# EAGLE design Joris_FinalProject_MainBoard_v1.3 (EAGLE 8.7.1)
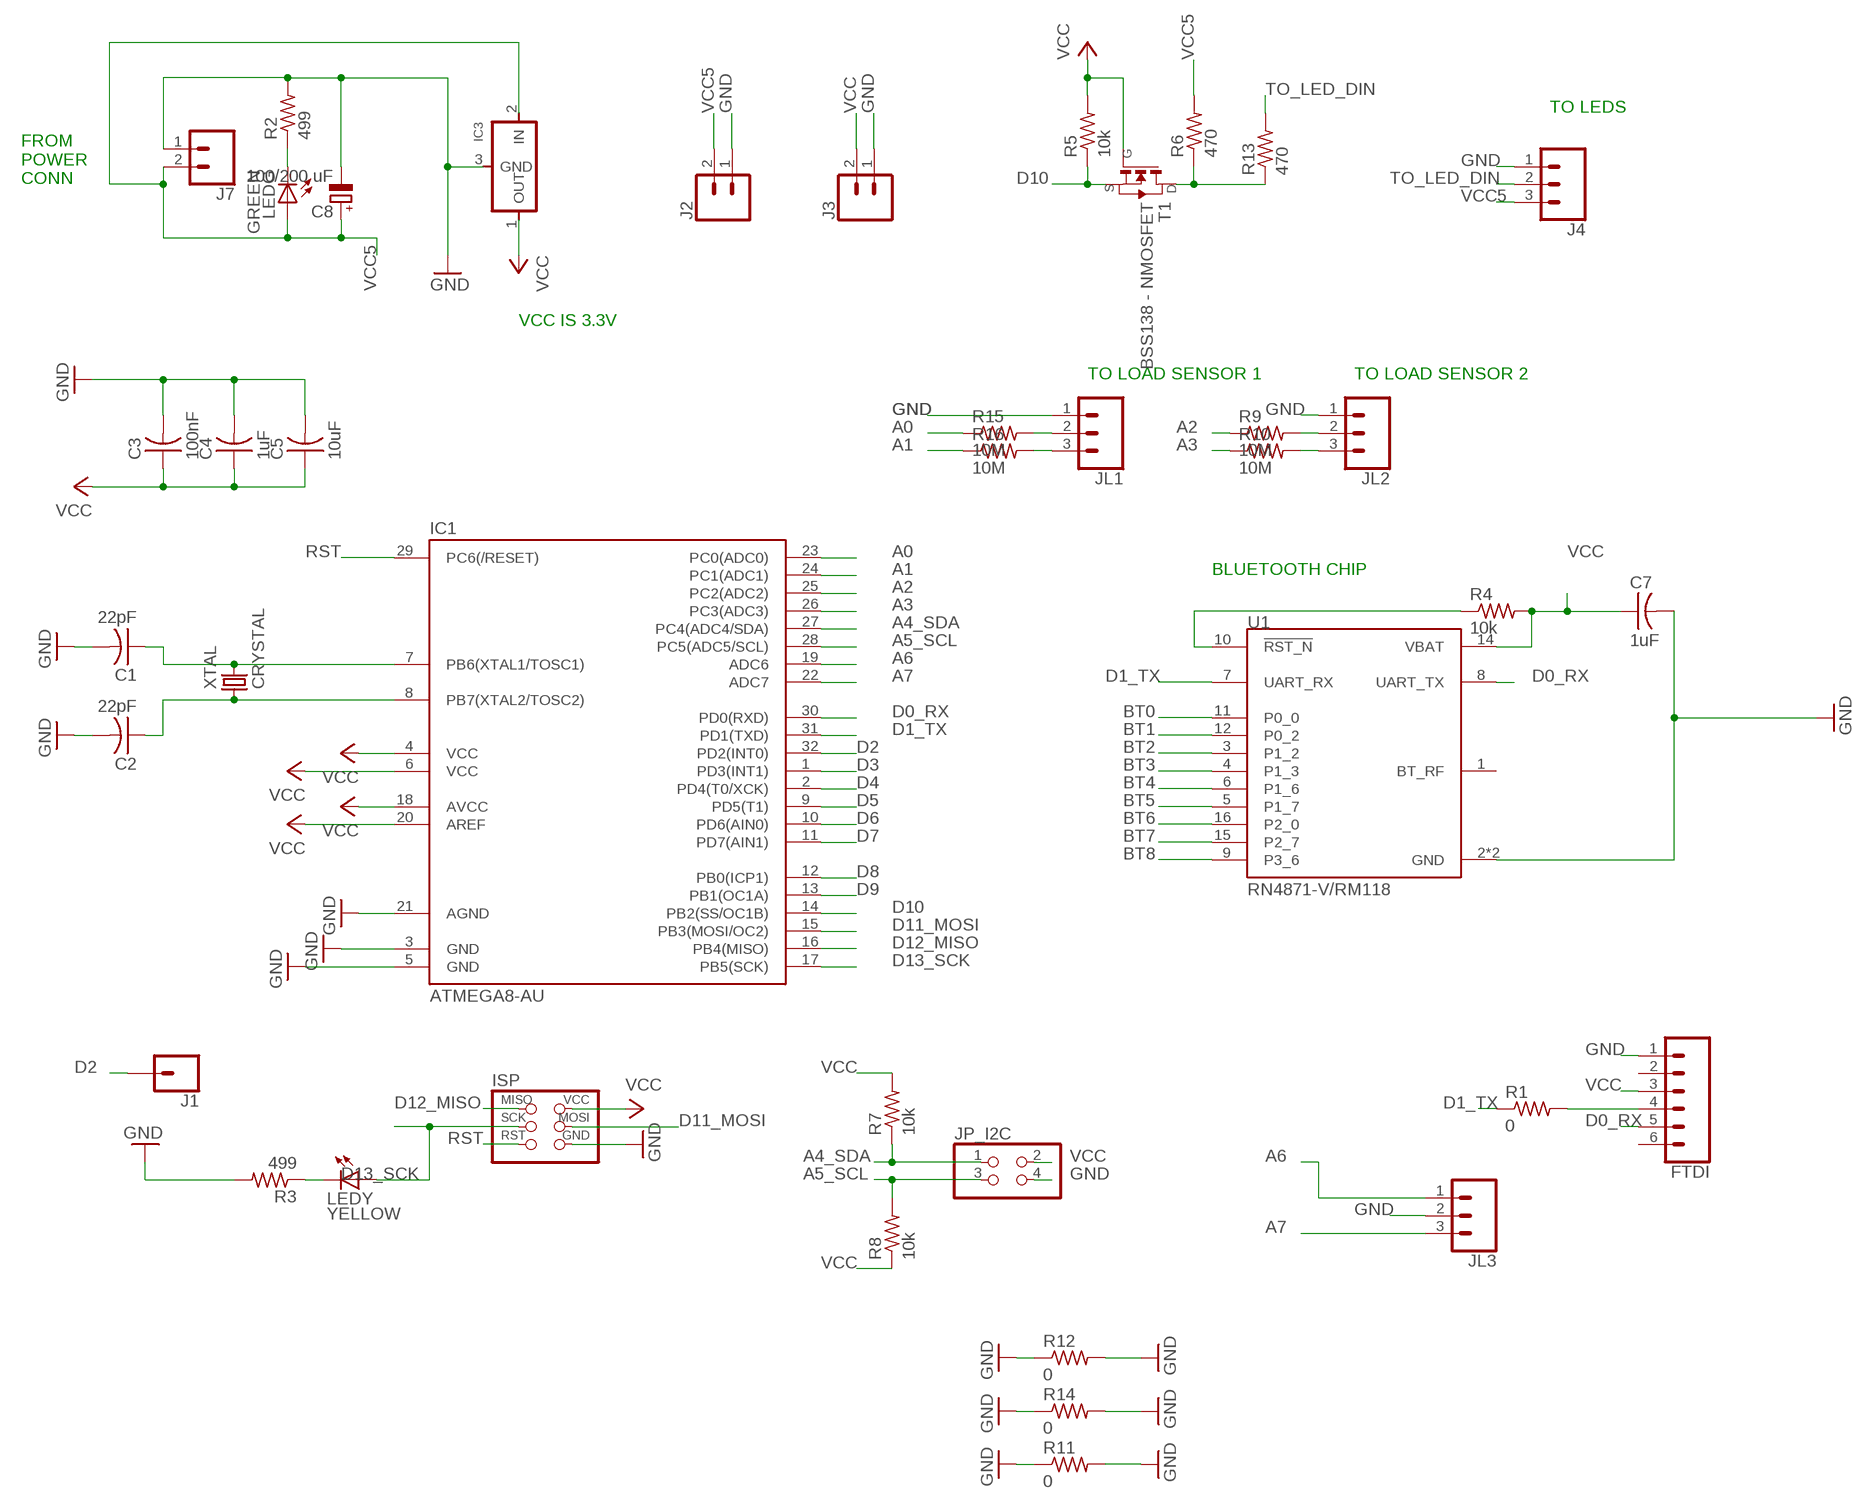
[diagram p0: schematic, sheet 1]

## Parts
C1  22pF  CAP-US1206FAB  [C1206FAB]
C2  22pF  CAP-US1206FAB  [C1206FAB]
C3  100nF  CAP-US1206FAB  [C1206FAB]
C4  1uF  CAP-US1206FAB  [C1206FAB]
C5  10uF  CAP-US1206FAB  [C1206FAB]
C7  1uF  CAP-US1206FAB  [C1206FAB]
C8  100/200 uF  CPOL-EUE3.5-8  [E3,5-8]
FTDI  CONN_06NO_SILK_NO_POP  [1X06_NO_SILK]
IC1  ATMEGA8-AU  [TQFP32-08]
IC3  REGULATORSOT23  [SOT23]
ISP  AVRISPSMD  [2X03SMD]
J1  CONN_01POGOPIN_HOLE_LARGE  [1X01_POGOPIN_HOLE_0.061_DIA]
J2  CONN_02JST-PTH-2  [JST-2-PTH]
J3  CONN_02JST-PTH-2  [JST-2-PTH]
J4  CONN_03JST-PTH-VERT  [JST-3-PTH-VERT]
J7  CONN_02JST-PTH-2  [JST-2-PTH]
JL1  CONN_03JST-PTH-VERT  [JST-3-PTH-VERT]
JL2  CONN_03JST-PTH-VERT  [JST-3-PTH-VERT]
JL3  CONN_03JST-PTH-VERT  [JST-3-PTH-VERT]
JP_I2C  PINHD-2X2-SMD  [2X02SMD]
LEDG  GREEN  LEDFAB1206  [LED1206FAB]
LEDY  YELLOW  LEDFAB1206  [LED1206FAB]
R1  0  RES-US1206FAB  [R1206FAB]
R2  499  RES-US1206FAB  [R1206FAB]
R3  499  RES-US1206FAB  [R1206FAB]
R4  10k  RES-US1206FAB  [R1206FAB]
R5  10k  RES-US1206FAB  [R1206FAB]
R6  470  RES-US1206FAB  [R1206FAB]
R7  10k  RES-US1206FAB  [R1206FAB]
R8  10k  RES-US1206FAB  [R1206FAB]
R9  10M  RES-US1206FAB  [R1206FAB]
R10  10M  RES-US1206FAB  [R1206FAB]
R11  0  RES-US1206FAB  [R1206FAB]
R12  0  RES-US1206FAB  [R1206FAB]
R13  470  RES-US1206FAB  [R1206FAB]
R14  0  RES-US1206FAB  [R1206FAB]
R15  10M  RES-US1206FAB  [R1206FAB]
R16  10M  RES-US1206FAB  [R1206FAB]
T1  BSS138 - NMOSFET  NMOSFETSOT23  [SOT-23]
U1  RN4871-V/RM118  [XCVR_RN4871-V/RM118]
XTAL  CRYSTAL  [2-SMD-5X3MM]

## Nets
A0: IC1.23(PC0(ADC0)) JL1.2 R15.1 R15.2
A1: IC1.24(PC1(ADC1)) JL1.3 R16.1 R16.2
A2: IC1.25(PC2(ADC2)) JL2.2 R9.1 R9.2
A3: IC1.26(PC3(ADC3)) JL2.3 R10.1 R10.2
A4_SDA: IC1.27(PC4(ADC4/SDA)) JP_I2C.1 R7.1
A5_SCL: IC1.28(PC5(ADC5/SCL)) JP_I2C.3 R8.2
A6: IC1.19(ADC6) JL3.1
A7: IC1.22(ADC7) JL3.3
BT0: U1.11(P0_0)
BT1: U1.12(P0_2)
BT2: U1.3(P1_2)
BT3: U1.4(P1_3)
BT4: U1.6(P1_6)
BT5: U1.5(P1_7)
BT6: U1.16(P2_0)
BT7: U1.15(P2_7)
BT8: U1.9(P3_6)
D0_RX: FTDI.5 IC1.30(PD0(RXD)) U1.8(UART_TX)
D1_TX: IC1.31(PD1(TXD)) R1.1 U1.7(UART_RX)
D2: IC1.32(PD2(INT0)) J1.1
D3: IC1.1(PD3(INT1))
D4: IC1.2(PD4(T0/XCK))
D5: IC1.9(PD5(T1))
D6: IC1.10(PD6(AIN0))
D7: IC1.11(PD7(AIN1))
D8: IC1.12(PB0(ICP1))
D9: IC1.13(PB1(OC1A))
D10: IC1.14(PB2(SS/OC1B)) R5.1 T1.2(S)
D11_MOSI: IC1.15(PB3(MOSI/OC2)) ISP.4(MOSI)
D12_MISO: IC1.16(PB4(MISO)) ISP.1(MISO)
D13_SCK: IC1.17(PB5(SCK)) ISP.3(SCK) LEDY.1(A)
GND: C1.2 C2.2 C3.2 C4.2 C5.2 C7.2 C8.- FTDI.1 IC1.3(GND) IC1.5(GND) IC1.21(AGND) IC3.3(GND) ISP.6(GND) J2.1 J3.1 J4.1 J7.1 JL1.1 JL2.1 JL3.2 JP_I2C.4 R2.2 R3.2 R11.1 R11.2 R12.1 R12.2 R14.1 R14.2 U1.2(GND) U1.13(GND)
N$1: LEDY.2(C) R3.1
N$5: LEDG.2(C) R2.1
N$6: C2.1 IC1.8(PB7(XTAL2/TOSC2)) XTAL.P$1
N$7: C1.1 IC1.7(PB6(XTAL1/TOSC1)) XTAL.P$2
N$8: FTDI.4 R1.2
N$12: R4.1 U1.10(!RST_N)
R$4: R6.1 R13.1 T1.1(D)
RST: IC1.29(PC6(/RESET)) ISP.5(RST)
TO_LED_DIN: J4.2 R13.2
VCC: C3.1 C4.1 C5.1 C7.1 FTDI.3 IC1.4(VCC) IC1.6(VCC) IC1.18(AVCC) IC1.20(AREF) IC3.1(OUT) ISP.2(VCC) J3.2 JP_I2C.2 R4.2 R5.2 R7.2 R8.1 T1.3(G) U1.14(VBAT)
VCC5: C8.+ IC3.2(IN) J2.2 J4.3 J7.2 LEDG.1(A) R6.2
Unconnected: FTDI.2 FTDI.6 U1.1(BT_RF)

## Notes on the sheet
- TO LEDS
- FROM
  POWER
  CONN
- VCC IS 3.3V
- TO LOAD SENSOR 1 | TO LOAD SENSOR 2
- BLUETOOTH CHIP

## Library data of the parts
C1-C5 C7 = fab:CAP-US
C8 = rcl:CPOL-EU: POLARIZED CAPACITOR, European symbol; SPICEPREFIX: C
FTDI = SparkFun-Connectors:CONN_06: Multi connection point. Often used as Generic Header-pin footprint for 0.1 inch spaced/style header connections On any of the 0.1 inch spaced packages, you can populate with these: Break Away Headers - Straight (PRT-00116) Break Away Male Headers - Right Angle (PRT-00553) Female Headers (PRT-00115)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
IC1 = atmega8:ATMEGA8
IC3 = fab:REGULATOR
ISP = fab:AVRISP
J1 = SparkFun-Connectors:CONN_01: Single connection point. Often used as Generic Header-pin footprint for 0.1 inch spaced/style header connections
J2 J3 J7 = SparkFun-Connectors_latest:CONN_02: Multi connection point. Often used as Generic Header-pin footprint for 0.1 inch spaced/style header connections; PROD_ID: CONN-09863; SKU: PRT-09914
J4 JL1-JL3 = SparkFun-Connectors_latest:CONN_03: Multi connection point. Often used as Generic Header-pin footprint for 0.1 inch spaced/style header connections On any of the 0.1 inch spaced packages, you can populate with these: Break Away Headers - Straight (PRT-00116) Break Away Male Headers - Right Angle (PRT-00553) Female Headers (PRT-00115)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; PROD_ID: CONN-13230
JP_I2C = fab:PINHD-2X2-SMD
LEDG LEDY = fab:LED: LED
R1-R16 = fab:RES-US: Resistor (US Symbol)
T1 = fab:NMOSFET: MOS FET
U1 = RN4871-V_RM118:RN4871-V/RM118: Bluetooth 4.2 BLE Module Shielded Antenna ASCII Interface 9x11.5mm; AVAILABILITY: Good; DESCRIPTION: Bluetooth 4.2 BLE Module Shielded Antenna ASCII Interface 9x11.5mm; MF: Microchip; MP: RN4871-V/RM118; PACKAGE: SMD-16 Microchip; PRICE: 7.65 USD
XTAL = fab:CRYSTAL

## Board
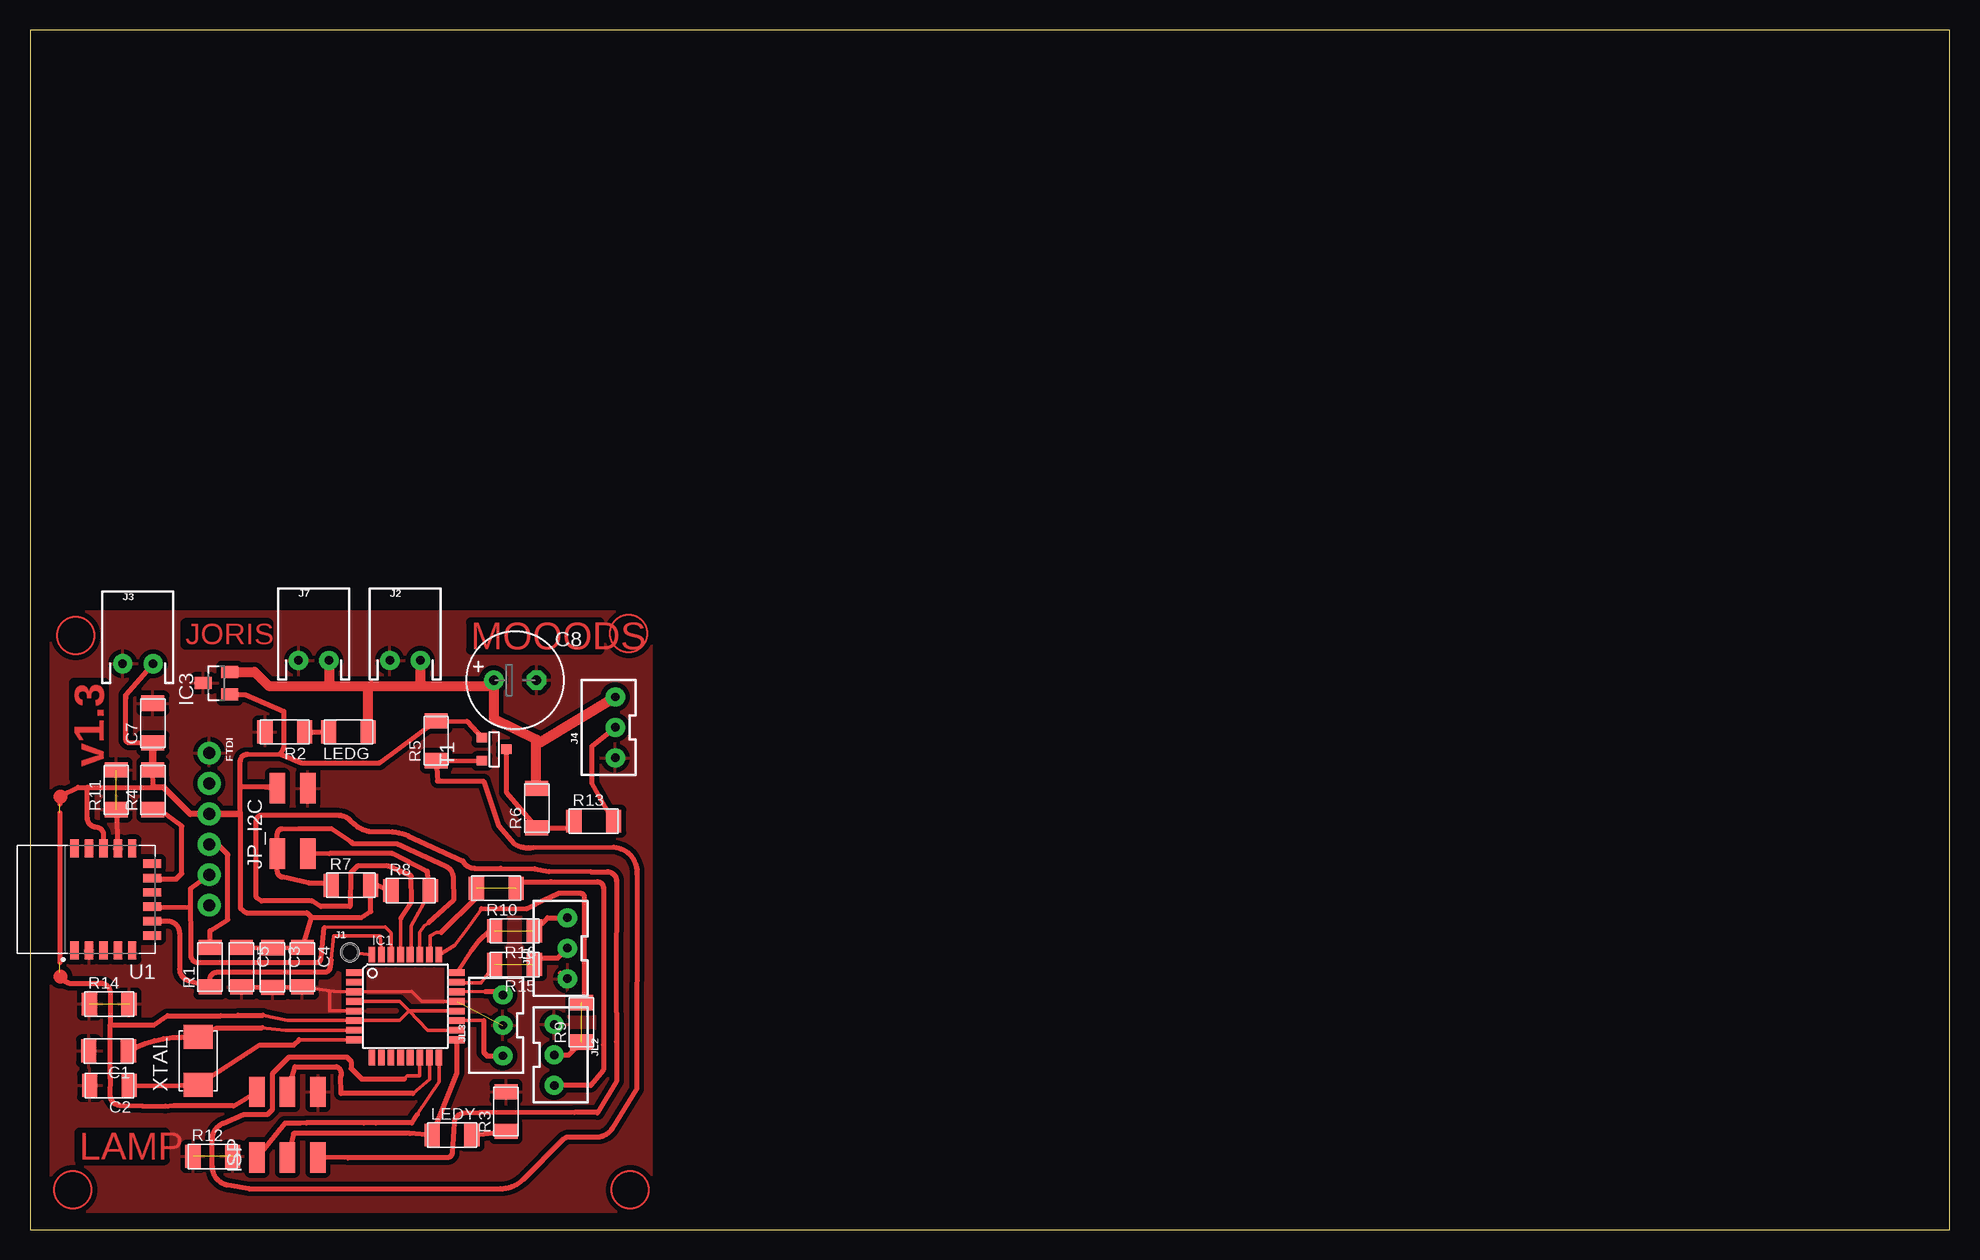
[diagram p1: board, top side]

Size 160 x 100 mm. Coordinates in mm from the lower left corner, seen from the top.
Outline: 0,0 160,0 160,100 0,100 0,0
Copper layers (1*16): Top 0.035mm / dielectric 1.5mm / Bottom 0.035mm
Design rules "default *": minimum track width 6mil, minimum drill 0.35mm, track to track 16mil, track to pad 16mil, pad to pad 16mil, via to via 16mil, smd to smd 16mil, copper to edge 40mil, drill to drill 16mil, minimum pad ring 10mil, minimum via ring 8mil, stop-mask expansion 4mil, vias tented up to drill 0mil, thermal gap 16mil

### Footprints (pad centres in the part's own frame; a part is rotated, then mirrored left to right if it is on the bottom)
C1206FAB = smd 1.27 x 1.905: 1 -1.651,0; 2 1.651,0
E3,5-8 = drill 0.813 pad 1.6: + -1.778,0 | drill 0.813 pad 1.6 octagon: - 1.778,0
1X06_NO_SILK = drill 1.016 pad 1.88: 1 0,0; 2 2.54,0; 3 5.08,0; 4 7.62,0; 5 10.16,0; 6 12.7,0
TQFP32-08 = smd 1.27 x 0.559: 1 -4.293,2.8; 2 -4.293,2; 3 -4.293,1.2; 4 -4.293,0.4; 5 -4.293,-0.4; 6 -4.293,-1.2; 7 -4.293,-2; 8 -4.293,-2.8; 17 4.293,-2.8; 18 4.293,-2; 19 4.293,-1.2; 20 4.293,-0.4; 21 4.293,0.4; 22 4.293,1.2; 23 4.293,2; 24 4.293,2.8 | smd 0.559 x 1.27: 9 -2.8,-4.293; 10 -2,-4.293; 11 -1.2,-4.293; 12 -0.4,-4.293; 13 0.4,-4.293; 14 1.2,-4.293; 15 2,-4.293; 16 2.8,-4.293; 25 2.8,4.293; 26 2,4.293; 27 1.2,4.293; 28 0.4,4.293; 29 -0.4,4.293; 30 -1.2,4.293; 31 -2,4.293; 32 -2.8,4.293
SOT23 = smd 1 x 1.4: 1 -0.95,-1.1; 2 0.95,-1.1; 3 0,1.1
2X03SMD = smd 2.54 x 1.27: 1 -2.54,2.54; 2 2.92,2.54; 3 -2.54,0; 4 2.92,0; 5 -2.54,-2.54; 6 2.92,-2.54
1X01_POGOPIN_HOLE_0.061_DIA = drill 0.9 pad 0.813: 1 0,0 | hole 1.549: 0,0
JST-2-PTH = drill 0.7 pad 1.6: 1 -1.27,0; 2 1.27,0
JST-3-PTH-VERT = drill 0.7 pad 1.6: 1 -2.54,-0.55; 2 0,-0.55; 3 2.54,-0.55
2X02SMD = smd 2.54 x 1.27: 1 -2.54,1.27; 2 2.92,1.27; 3 -2.54,-1.27; 4 2.92,-1.27
LED1206FAB = smd 1.27 x 1.905: 1 -1.651,0; 2 1.651,0
R1206FAB = smd 1.27 x 1.905: 1 -1.651,0; 2 1.651,0
SOT-23 = smd 0.787 x 0.889: 1 0.025,-1.016; 2 -0.94,1.016; 3 0.991,1.016
XCVR_RN4871-V/RM118 = smd 1.5 x 0.7: 1 -4.25,0.95; 2 -4.25,-0.25; 3 -4.25,-1.45; 4 -4.25,-2.65; 5 -4.25,-3.85; 12 4.25,-3.85; 13 4.25,-2.65; 14 4.25,-1.45; 15 4.25,-0.25; 16 4.25,0.95 | smd 0.7 x 1.5: 6 -3,-5.5; 7 -1.8,-5.5; 8 -0.6,-5.5; 9 0.6,-5.5; 10 1.8,-5.5; 11 3,-5.5
2-SMD-5X3MM = smd 2 x 2.4: P$1 -2,0; P$2 2,0

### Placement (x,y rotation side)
C1  6.55,14.88 180 top
C2  6.63,12.01 180 top
C3  20.22,21.84 270 top
C4  22.71,21.87 270 top
C5  17.63,21.87 270 top
C7  10.24,42.21 90 top
C8  40.44,45.8 0 top
FTDI  14.94,39.73 270 top
IC1  31.29,18.62 0 top
IC3  15.54,45.54 90 top
ISP  21.46,8.56 90 top
J1  26.67,23.11 0 top
J2  31.27,47.45 0 top
J3  8.99,47.17 0 top
J4  48.23,41.86 90 top
J7  23.65,47.45 0 top
JL1  44.25,23.44 90 top
JL2  44.25,14.55 270 top
JL3  38.86,17.02 90 top
JP_I2C  21.89,33.86 90 top
LEDG  26.54,41.48 180 top
LEDY  35.18,7.87 0 top
R1  15.01,21.87 90 top
R2  21.23,41.48 180 top
R3  39.67,9.83 90 top
R4  10.24,36.65 90 top
R5  33.86,40.74 90 top
R6  42.24,35.13 90 top
R7  26.75,28.7 0 top
R8  31.72,28.24 0 top
R9  45.97,17.27 90 top
R10  38.86,28.45 180 top
R11  7.19,36.65 90 top
R12  15.24,6.1 0 top
R13  46.99,34.04 0 top
R14  6.6,18.8 0 top
R15  40.39,22.1 180 top
R16  40.39,24.89 180 top
T1  38.68,40.01 90 top
U1  4.67,27.51 90 top
XTAL  14.02,14.05 90 top

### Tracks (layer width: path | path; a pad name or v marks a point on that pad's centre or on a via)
A0  (1 unrouted)
  Top 0.305: IC1.23 35.63,20.57 37.59,20.57 R15.2
  Top 0.406: JL1.2 43.98,22.63 42.57,22.63 R15.1 | 38.73,21.46 R15.2
A1  (1 unrouted)
  Top 0.305: IC1.24 36.79,23.27
  Top 0.406: 36.79,23.27 37.5,24.13 38.26,24.89 R16.2 | R16.1 43.13,25.98 JL1.3
A2  (1 unrouted)
  Top 0.305: IC1.25 35.41,23.7 36.35,24.94 37.64,26.75
  Top 0.406: 37.64,26.75 39.22,26.77 41.38,26.75 42.95,27.51 44.02,28.02 45.9,28.02 arc-90 46.23,27.69 46.23,19.18 R9.2 | JL2.2 44.91,14.55 R9.1
A3  (1 unrouted)
  Top 0.305: IC1.26 33.36,22.97 33.36,24.5 33.9,24.77 34.29,24.77 34.38,24.77
  Top 0.406: JL2.3 46.75,12.01 47.8,13.32 47.8,15.42 47.8,28.48 arc90 47.3,28.98 43.44,28.98 43.43,28.97 43.37,28.98 41.05,28.98 R10.1 | 34.29,24.77 37.21,27.69 R10.2
A4_SDA
  Top 0.305: IC1.27 32.49,24.77 32.87,25.3 33.25,25.58
  Top 0.406: 33.25,25.58 35.31,27.45 35.28,29.3 arc65 34.63,30.3 30.56,32.18 26.9,32.18 26.72,32.33 25.12,33.43 22.43,33.43 21.01,33.41 arc89 20.62,33.02 JP_I2C.1 20.62,29.87 arc78 21.02,29.38 23.19,28.91 24.89,28.91 R7.1
A5_SCL
  Top 0.305: IC1.28 31.76,22.97 31.76,24.14 31.75,25.32 R8.2
  Top 0.406: R8.2 33.12,29.87 30.23,31.34 24.97,31.34 JP_I2C.3
A6
  Top 0.305: IC1.19 36.75,17.42 37.82,17.42
  Top 0.406: 37.82,17.42 37.82,14.76 38.1,14.48 JL3.1
A7
  Top 0.305: IC1.22 37.97,19.84
  Top 0.406: 37.97,19.84 39.13,19.84 JL3.3
D0_RX
  Top 0.305: IC1.30 30.09,24.75 29.6,25.21 24.54,25.18
  Top 0.406: U1.8 10.15,26.88 13.38,26.86 | 24.54,25.18 24.25,22.6 arc-84 23.87,22.25 17.16,22.25 14.03,22.25 arc-90 13.4,22.88 13.4,24.51 13.36,26.91 13.38,26.86 | 13.38,26.86 13.38,28.42 FTDI.5
D1_TX
  Top 0.305: IC1.31 29.18,24.49 25.32,24.46 25.09,22.5
  Top 0.406: U1.7 11.5,25.7 arc-89 12.47,24.72 12.48,21.7 arc73 13.18,20.77 R1.1 15,20.86 arc-91 15.56,21.44 24.54,21.44 arc83 25.02,21.86 25.09,22.5
D2
  Top 0.305: J1.1 IC1.32
D10
  Top 0.305: 31.19,12.55 31.45,12.8 32.46,12.8 32.49,12.83 IC1.14
  Top 0.406: T1.2 R5.1 33.96,37.39 37.8,37.39 39.06,33.63 40.34,32.15 arc42 41.95,31.85 48.68,31.88 arc-90 50.59,29.61 50.55,11.68 48.56,8.46 arc-58 47.24,7.72 44.96,7.72 arc45 44.44,7.51 41.13,4.2 arc-45 39.21,3.4 18.24,3.4 16.51,3.69 arc-81 15.19,5.25 15.19,7.49 arc-67 16.11,8.87 17.83,9.6 19.81,9.6 20.22,10.01 20.22,13 21.59,14.38 21.89,14.38 22.09,14.39 22.21,14.38 22.22,14.38 26.4,14.38 26.76,14.03 26.76,13.43 27.64,12.55 31.19,12.55
D11_MOSI
  Top 0.305: IC1.15 33.29,12.54 31.93,11.35
  Top 0.406: 31.93,11.35 25.93,11.35 25.91,12.78 arc88 25.55,13.57 22.1,13.56 ISP.4
D12_MISO
  Top 0.305: 32.28,9.6 34.09,12.3 IC1.16
  Top 0.406: 32.28,9.6 31.83,8.89 28.84,8.89 27.84,8.88 23.02,8.88 22.53,8.87 21.23,8.87 ISP.1
D13_SCK
  Top 0.406: IC1.17 35.59,13.08 LEDY.1 31.65,8 21.97,8 ISP.3
GND  (4 unrouted)
  Top 0.305: IC1.21 32.64,19.02 31.8,19.84 IC1.3 25.3,19.84 25,19.89 | 25,19.89 C4.2 | IC1.5 24.99,18.21 25,19.89
  Top 0.406: C5.2 C3.2 C4.2 | 44.22,21.36 JL1.1 | R11.1 U1.13
  pour Top: 1.78,51.51 51.77,51.51 51.77,1.5 1.78,1.47
N$1
  Top 0.406: LEDY.2 R3.1
N$5
  Top 0.406: R2.1 LEDG.2
N$6
  Top 0.305: 22.42,15.82 IC1.8
  Top 0.406: C2.1 11.03,11.99 XTAL.P$1 19.16,15.39 21.99,15.39 22.42,15.82
N$7
  Top 0.305: 19.36,16.82 19.3,16.82 21.26,16.61 23.81,16.62 IC1.7
  Top 0.406: C1.1 arc-29 12.65,16.04 XTAL.P$2 15.57,16.81 19.36,16.82
N$8
  Top 0.406: R1.2 15.01,24.91 16.48,25.82 16.48,31.22 16.51,31.24 15.65,32.11 FTDI.4
N$12
  Top 0.406: 10.12,29.31 U1.10 10.78,29.21 12.19,29.21 12.65,29.67 12.65,33.63 10.77,35 R4.1
R$4
  Top 0.406: T1.1 39.7,36.45 R6.1 45.29,33.48 R13.1
RST
  Top 0.305: IC1.29 30.89,25.66 30.91,25.93
  Top 0.406: 30.91,25.93 31.8,27.33 31.77,29.46 29.82,30.3 27.3,30.3 26.72,29.72 26.67,26.92 24.23,26.92 23.52,27.38 19.28,27.38 18.87,27.69 18.87,34.11 arc-90 19.3,34.54 25.65,34.54 arc-42 26.65,34.16 27.07,33.77 arc42 28.61,33.17 29.91,33.17 arc-25 31.53,32.82 36.07,30.73 36.12,30.64 arc60 37.03,30.12 39.23,30.12 42.08,30.07 43.26,29.83 46.81,29.81 48.14,29.82 arc-90 48.89,29.07 48.87,20.5 48.9,15.67 48.9,12.34 47.3,9.73 47.27,9.75 45.39,9.75 37.44,9.73 36.19,9.7 arc85 35.36,8.9 35.2,6.4 arc-86 34.77,5.99 26.49,5.97 ISP.5
TO_LED_DIN
  Top 0.406: J4.2 46.85,40.31 46.85,37.2 R13.2
VCC  (2 unrouted)
  Top 0.305: IC1.20 31.62,18.22 | 31.62,18.22 30.81,19.02 30.8,19.02 IC1.4 | 31.62,18.22 30.82,17.42 IC1.6 21.42,17.42 19.43,17.86 | 29.01,28.65 R7.2 | 31.62,18.22 33.15,16.61 IC1.18
  Top 0.406: T1.3 36.42,42.37 R5.2 29.13,38.91 22.63,38.91 20.85,39.65 | IC3.1 17.95,44.6 21.18,43.2 21.18,40.45 arc-33 21.03,39.91 20.85,39.65 | C5.1 C3.1 C4.1 23.44,26.01 | R8.1 29.01,28.65 | ISP.2 16.94,10.29 16.88,10.35 11.98,10.35 11.28,10.29 9.37,10.31 7.47,10.37 arc-89 6.66,11.21 6.68,12.62 6.68,17.04 | 6.68,17.04 10.34,17.04 11.46,17.83 15.9,17.83 17.35,17.86 19.43,17.86 | J3.2 7.97,44.55 | 7.97,44.55 7.98,44.22 | C7.1 8.31,40.56 arc-90 7.98,40.89 7.98,44.55 7.97,44.55 | 4.78,36.85 4.01,36.85 2.49,36.09 2.49,35.46 | 4.78,36.85 10.26,36.85 R4.2 | 23.44,26.01 23.44,26.06 23.09,26.42 18.03,26.42 17.53,26.8 17.53,34.75 | 20.85,39.65 18.12,39.62 arc90 17.53,39.03 17.53,36.93 | 19.2,36.93 JP_I2C.2 19.86,36.93 17.53,36.93 | 23.44,26.01 27.64,26.01 28.4,26.52 R7.2 | U1.14 6.13,33.03 arc69 5.53,33.54 5.45,33.55 arc-83 4.78,34.31 4.78,36.85 | 6.68,17.04 6.68,19.88 arc90 5.79,20.52 3.47,20.51 arc-75 2.49,21.39 2.49,21.44 | 17.42,34.65 17.53,34.75 | 17.53,34.75 17.53,36.93 | 2.49,34.75 2.49,22.25
  Top 0.508: FTDI.3 17.42,34.65 17.5,34.57 17.5,34.54 17.4,34.65 FTDI.3 | FTDI.3 13.36,34.65 11.15,36.85 10.26,36.85
  Top 0.61: C7.1 R4.2
VCC5
  Top 0.813: IC3.2 18.71,46.49 19.89,45.31 25.15,45.31 | 25.15,45.31 28.45,45.31 | 28.45,45.31 32.51,45.31 | 32.51,45.31 38.18,45.31 C8.+ 38.66,42.62 42.16,40.89 | J2.2 32.54,45.34 32.51,45.31 | J7.2 24.92,45.54 25.15,45.31 | LEDG.1 28.19,45.06 28.45,45.31 | 42.16,40.89 42.16,36.85 R6.2 | 42.16,40.89 42.47,40.59 J4.3
(copper drawn outside any net)
  shapes: Top circle x6

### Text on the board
Top: JORIS | MOOODS | v1.3 | LAMP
